PROGRAM MAIN
VAR
	power1:MC_Power;
	axis1: AXIS_REF;
	power_do: BOOL;
	jog1:MC_Jog;
	jog_for: BOOL;
	jog_back: BOOL;
	gearin:mc_gearin;
	gearout:mc_gearout;
	power2:mc_power;
	axis2:axis_ref;
	gearin_do:BOOL;
	gearout_do:bool;
END_VAR

power1(
	Axis:=axis1 , 
	Enable:=power_do , 
	Enable_Positive:=TRUE , 
	Enable_Negative:= TRUE, 
	Override:= , 
	BufferMode:= , 
	Options:= , 
	Status=> , 
	Busy=> , 
	Active=> , 
	Error=> , 
	ErrorID=> );
jog1(
	Axis:=axis1 , 
	JogForward:=jog_for , 
	JogBackwards:= jog_back, 
	Mode:= , 
	Position:= , 
	Velocity:= , 
	Acceleration:= , 
	Deceleration:= , 
	Jerk:= , 
	Done=> , 
	Busy=> , 
	Active=> , 
	CommandAborted=> , 
	Error=> , 
	ErrorID=> );
gearin(
	Master:= axis1, 
	Slave:=axis2 , 
	Execute:= gearin_do, 
	RatioNumerator:=1 , 
	RatioDenominator:=1 , 
	Acceleration:= , 
	Deceleration:= , 
	Jerk:= , 
	BufferMode:= , 
	Options:= , 
	InGear=> , 
	Busy=> , 
	Active=> , 
	CommandAborted=> , 
	Error=> , 
	ErrorID=> );
gearout(
	Slave:=axis2 , 
	Execute:=gearout_do , 
	Options:= , 
	Done=> , 
	Busy=> , 
	Error=> , 
	ErrorID=> );

END_PROGRAM
